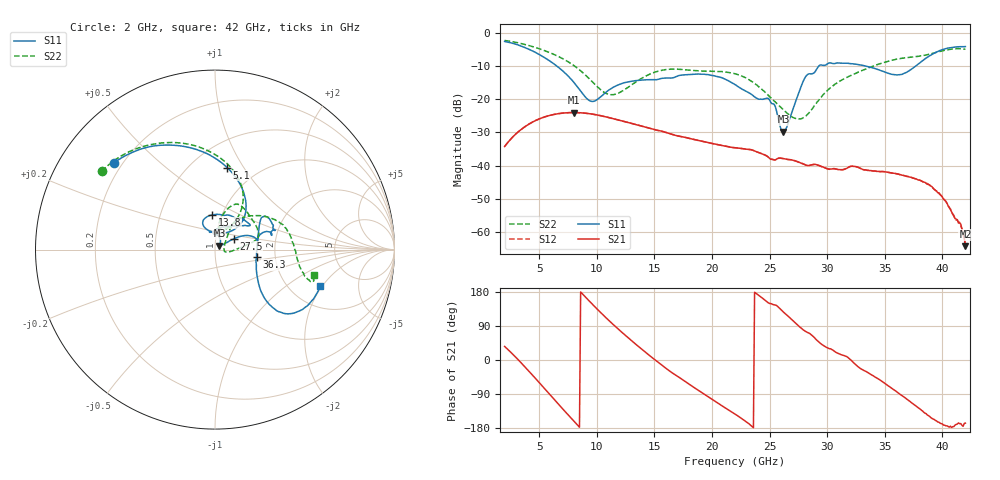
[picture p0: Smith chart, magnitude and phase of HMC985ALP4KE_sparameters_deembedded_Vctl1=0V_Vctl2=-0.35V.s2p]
!s2p File: Measurements: S11, S21, S12, S22
# GHz S dB R 50.0
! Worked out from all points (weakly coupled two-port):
!   401 points, 2 GHz to 42 GHz, reference 50 ohm
!   highest |S21| = -24.01 dB at 8 GHz (marker M1); lowest = -64.3 dB at 42 GHz (marker M2)
!   lowest |S11| = -29.8 dB at 26.2 GHz (marker M3), VSWR 1.07, Z = 52.5 + j2.22 ohm
!   |S11| at or under -10 dB: 6.532 GHz to 29.27 GHz (22.74 GHz wide, 127 % of centre); 33.34 GHz to 37.69 GHz (4.348 GHz wide, 12.2 % of centre)
!   |S22| runs from -26.0 to -2.3 dB; largest |S21 - S12| = 0.00016
!   S11 on the Smith chart (normalised r, x): 2 GHz: 0.17, +0.36; 5.1 GHz: 0.73, +0.85; 13.8 GHz: 0.90, +0.36; 27.5 GHz: 1.22, +0.15; 36.3 GHz: 1.59, -0.14; 42 GHz: 2.90, -1.91
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2  -2.58 139.5  -34.24 35.9  -34.25 35.9  -2.29 145.3
3.5  -4.08 111.6  -28.94 -9.6  -28.94 -9.6  -3.28 121.5
5.1  -6.70 81.6  -25.79 -62.9  -25.80 -62.9  -4.90 97.1
8  -14.87 45.0  -24.01 -160.9  -24.02 -161.0  -9.81 60.8
8.7  -18.01 51.6  -24.11 176.2  -24.11 176.2  -11.73 56.3
9.7  -20.65 86.9  -24.52 144.6  -24.53 144.6  -15.04 55.3
11.2  -16.90 115.7  -25.65 100.0  -25.66 100.0  -18.63 71.2
13.8  -14.26 95.3  -28.00 31.1  -28.00 31.1  -13.90 77.0
15.4  -13.94 73.0  -29.45 -7.2  -29.45 -7.2  -11.47 68.3
19.4  -12.51 34.7  -32.87 -91.7  -32.87 -91.8  -11.54 34.7
22  -15.57 52.2  -34.61 -142.4  -34.61 -142.5  -12.32 14.3
25  -20.23 97.6  -37.82 149.2  -37.82 149.2  -19.19 -1.1
26.2  -29.81 40.9  -37.87 126.6  -37.89 126.6  -23.18 -11.8
27.5  -18.42 29.6  -38.93 90.2  -38.93 90.2  -25.96 -0.4
28.1  -13.37 20.7  -39.75 75.9  -39.72 75.8  -25.23 19.2
28.7  -12.32 12.8  -39.73 64.7  -39.72 64.7  -22.88 35.6
31.1  -9.13 24.1  -41.20 15.7  -41.22 15.5  -14.53 54.5
35.4  -12.27 12.4  -42.05 -70.1  -42.08 -70.4  -8.48 25.6
36.3  -12.57 -10.1  -42.70 -90.2  -42.69 -89.9  -7.80 17.8
39.8  -5.31 -41.3  -48.71 -166.6  -48.66 -166.6  -5.56 -16.6
41.5  -4.18 -23.0  -57.27 -168.1  -57.08 -167.4  -4.76 -17.4
42  -4.14 -19.0  -64.26 -166.6  -63.65 -164.5  -4.91 -14.5
